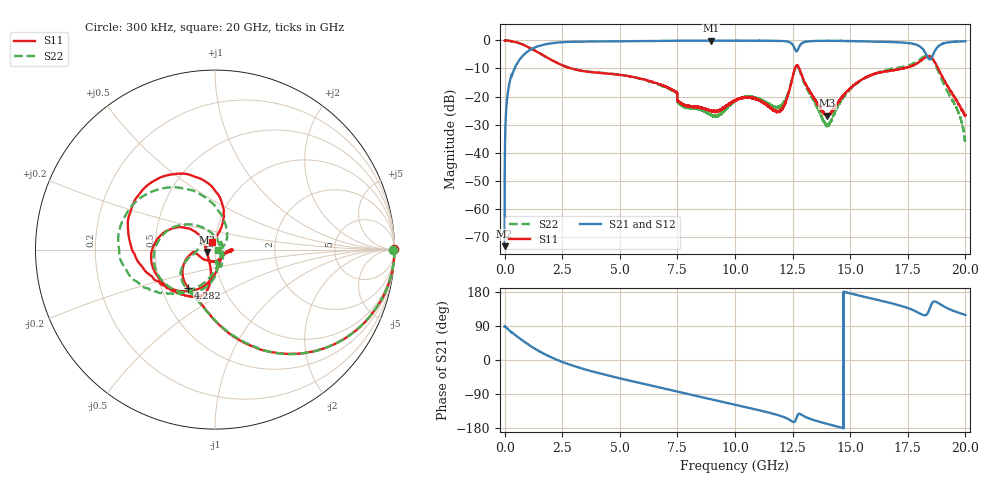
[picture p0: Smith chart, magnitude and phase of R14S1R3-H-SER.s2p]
!{R14S1R3}
!Johanson Technology Inc.
!www.johansontechnology.com
!Test Board Conditions:
!Substrate Type  RO4350B
!Substrate Thickness  20 mil
!Substrate Dk  3.66
!TL Type: GCPW
!TL Trace Width  36 mil
!TL Gap  12 mil
!Electrode orientation  Horizontal
!DUT TOPOLOGY	SERIES
!Mounting Pad LxW  26x36 mil
! Created Fri Jan  8 21:45:55 2021
# hz S ma R 50
! 2 Port Network Data from SP1.SP block
! freq  magS11  angS11  magS21  angS21  magS12  angS12  magS22  angS22
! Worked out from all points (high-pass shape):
!   20001 points, 300 kHz to 20 GHz, reference 50 ohm
!   highest |S21| = -0.05 dB at 8.963 GHz (marker M1); lowest = -73.4 dB at 300 kHz (marker M2)
!   |S21| within 3 dB of the highest: 1.175 GHz to 12.6 GHz (11.42 GHz wide, 166 % of centre); 12.74 GHz to 18.15 GHz (5.409 GHz wide, 35 % of centre)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
!   lowest |S11| = -26.8 dB at 14.01 GHz (marker M3), VSWR 1.10, Z = 45.8 - j1.21 ohm
!   |S11| at or under -10 dB: 2.899 GHz to 12.6 GHz (9.699 GHz wide, 125 % of centre); 12.79 GHz to 17.29 GHz (4.503 GHz wide, 29.9 % of centre); 18.82 GHz to end of sweep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
!   |S22| runs from -37.2 to 0.0 dB; largest |S21 - S12| = 0.018
!   S11 on the Smith chart (normalised r, x): 300 kHz: open; 4.282 GHz: 0.68, -0.31; 20 GHz: 0.97, +0.08
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300000  0.9951 0.1  0.0002147 87.4  0.0002819 111.8  0.9923 -0.0
1.013e8  0.9962 -5.9  0.08467 84.1  0.08511 84.0  0.9959 -5.8
1.333e8  0.9936 -7.6  0.1112 82.3  0.1117 82.2  0.9928 -7.6
5.143e8  0.9259 -26.1  0.3703 63.4  0.3714 63.6  0.9251 -26.1
1.8323e9  0.4996 -77.4  0.862 12.7  0.8632 12.7  0.498 -77.0
3.3343e9  0.2878 -111.3  0.9535 -22.1  0.954 -22.0  0.2898 -112.5
4.2823e9  0.2602 -125.2  0.9602 -37.7  0.9612 -37.8  0.2636 -129.9
6.6673e9  0.1691 -161.3  0.9814 -71.7  0.981 -71.7  0.1646 -160.6
8.9633e9  0.05664 -51.7  0.9944 -103.7  0.9929 -103.8  0.04739 26.5
1.00003e10  0.08586 -1.8  0.9897 -117.8  0.9887 -117.9  0.08333 -60.9
1.19623e10  0.05591 -47.2  0.9781 -147.3  0.9809 -147.3  0.06756 -82.2
1.24073e10  0.1532 -94.0  0.9158 -159.3  0.9189 -159.1  0.1597 -92.1
1.26843e10  0.3608 -163.1  0.6409 -150.2  0.6438 -150.4  0.3493 -162.4
1.33343e10  0.1081 138.4  0.9735 -156.9  0.9717 -156.9  0.09603 103.3
1.40123e10  0.0455 -163.2  0.9837 -168.8  0.9858 -168.8  0.03165 6.2
1.50633e10  0.1471 -99.3  0.9734 174.8  0.9745 174.6  0.1447 -97.5
1.66673e10  0.2827 -113.0  0.9423 151.5  0.9342 151.3  0.3037 -127.0
1.79803e10  0.4114 -164.8  0.8015 124.3  0.7899 123.9  0.4402 -151.0
1.84833e10  0.5126 131.8  0.4616 140.9  0.4584 141.4  0.5182 150.0
1.89703e10  0.237 78.8  0.8617 144.7  0.8627 144.5  0.2021 80.8
1.96953e10  0.07319 83.0  0.9585 125.0  0.9553 125.1  0.05187 23.1
2e10  0.04618 109.6  0.9663 118.9  0.9651 118.9  0.01381 -2.6
